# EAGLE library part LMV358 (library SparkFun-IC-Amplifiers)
IC LMV358 DUAL OP AMP Jellybean rail-to-rail output op-amp SparkFun Products SparkFun PicoBoard (WIG-11888) SparkFun Vernier Interface Shield (DEV-12858) SparkFun Blynk Board - ESP8266 (WRL-13794) SparkFun Digital Sandbox (DEV-12651 RoHS)
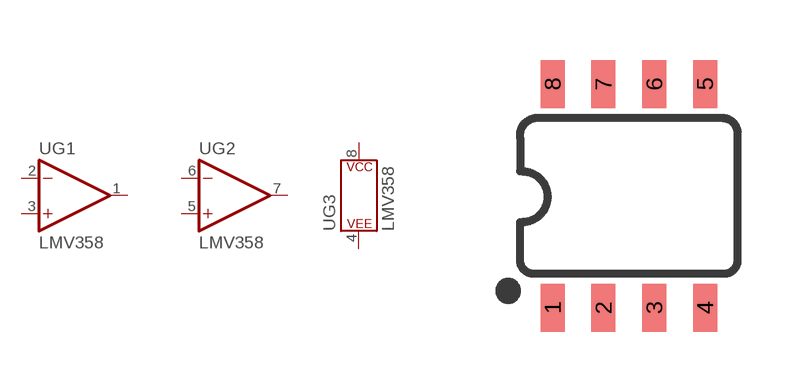
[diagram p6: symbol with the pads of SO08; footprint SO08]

Designator prefix U; gates G1=OP-AMP G2=OP-AMP G3=POWER_CONSORT

## LMV358SOIC (PROD_ID: IC-09657; VALUE: LMV358)  [SO08]
1  G1:OUT  out
2  G1:-IN  in
3  G1:+IN  in
4  G3:P$V-
5  G2:+IN  in
6  G2:-IN  in
7  G2:OUT  out
8  G3:P$V+

## Footprint SO08 (pad centres in mm)
SOIC, 0.15 inch width
smd 0.6 x 1.2: 1 -1.905,-2.8; 2 -0.635,-2.8; 3 0.635,-2.8; 4 1.905,-2.8; 5 1.905,2.8; 6 0.635,2.8; 7 -0.635,2.8; 8 -1.905,2.8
